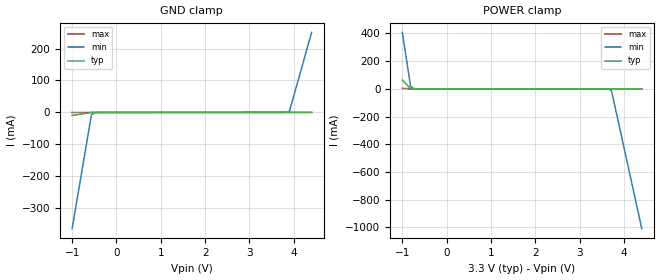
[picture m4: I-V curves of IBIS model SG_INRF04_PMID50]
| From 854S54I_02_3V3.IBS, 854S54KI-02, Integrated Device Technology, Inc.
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[Model]   SG_INRF04_PMID50
Model_type   Input
Polarity   Non-Inverting
Vinl = 0.8V
Vinh = 2.0V
|   typ   min   max
C_comp   2pF   1.5pF   2.5pF
|   typ   min   max
[Voltage range]   3.3V   3.135V   3.465V
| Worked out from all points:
|   GND clamp passes 1 mA (typ) near -0.60 V on its own axis
|   POWER clamp passes 1 mA (typ) near -0.78 V on its own axis
[GND_clamp]
|Voltage   I (typ)   I (min)   I (max)
-999mV    -9.476mA   -364.1mA   -125.5uA
-564.6mV  -216.6uA   -7.95mA    -85.05uA
-502.5mV  -96.27uA   -1.137mA   -82.6uA
-378.4mV  -79.91uA   -97.93uA   -78.01uA
3.841V    86.29uA    728.2uA    77.94uA
3.904V    89.26uA    4.844mA    80.23uA
4.4V      156.1uA    250.6mA    98.58uA
[Power_clamp]
|Voltage   I (typ)   I (min)   I (max)
-999mV    63.29mA    407.1mA    3.228mA
-812.8mV  2.097mA    20.04mA    143uA
-750.8mV  273.2uA    2.764mA    94uA
3.593V    -76.47uA   -333uA     -68.76uA
3.655V    -78.95uA   -1.957mA   -71.06uA
3.717V    -81.77uA   -14.07mA   -73.35uA
4.4V      -155.8uA   -1.009A    -98.58uA
